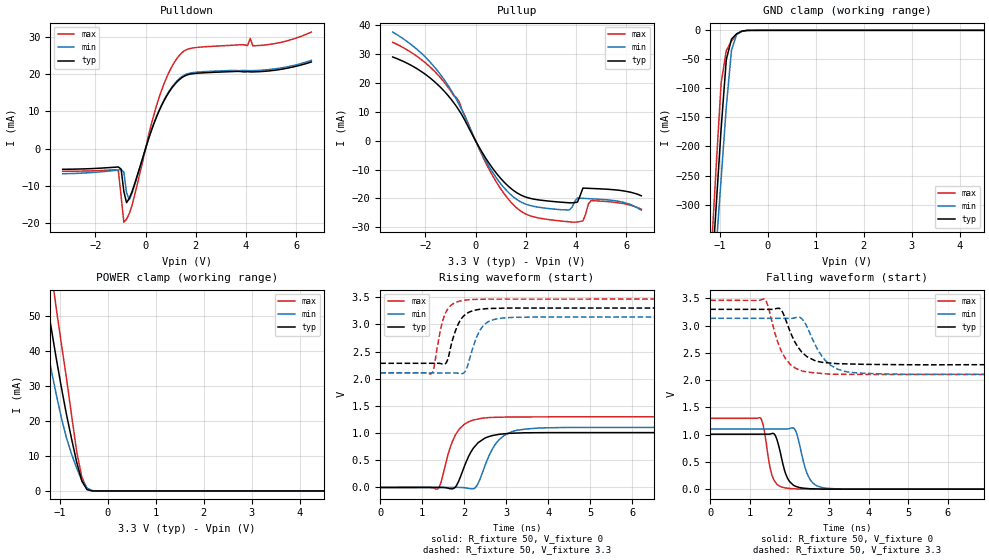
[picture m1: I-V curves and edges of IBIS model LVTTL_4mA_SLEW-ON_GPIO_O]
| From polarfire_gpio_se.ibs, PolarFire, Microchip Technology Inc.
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|   Model LVTTL_4mA_SLEW-ON_GPIO_O
[Model]   LVTTL_4mA_SLEW-ON_GPIO_O
Model_type   Output
Polarity   Non-Inverting
Enable   Active-High
Vmeas =   1.65
Cref =   5p
Rref =   1M
|   typ   min   max
C_comp_pullup   2.605e-12   2.605e-12   2.76e-12
C_comp_pulldown  2.605e-12   2.605e-12   2.76e-12
[Temperature Range]  25C   100C   -40C
[Voltage Range]  3.3   3.135   3.465
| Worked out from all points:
|   slope of the pulldown table from 0 to 0.495 V, typ, clamps not added: 52.5 ohm
|   slope of the pullup table from 0 to 0.495 V, typ, clamps not added: 68.4 ohm
|   GND clamp passes 1 mA (typ) near -0.51 V on its own axis
|   POWER clamp passes 1 mA (typ) near -0.46 V on its own axis
|   rising waveform, R_fixture 50, V_fixture 0: 20-80 % time 399ps typ, 429ps min, 348ps max; typ from 0 V to 1.01 V
|   rising waveform, R_fixture 50, V_fixture 3.3: 20-80 % time 275ps typ, 299ps min, 229ps max; typ from 2.28 V to 3.3 V
|   falling waveform, R_fixture 50, V_fixture 0: 20-80 % time 226ps typ, 254ps min, 186ps max; typ from 1.01 V to 0 V
|   falling waveform, R_fixture 50, V_fixture 3.3: 20-80 % time 444ps typ, 505ps min, 403ps max; typ from 3.3 V to 2.28 V
[GND Clamp]
| Voltage   I(typ)   I(min)   I(max)
-3.3V     -3.213A    -2.957A    -3.542A
-1.191V   -450mA     -505.3mA   -401.1mA
-1.083V   -310.2mA   -380.8mA   -242.7mA
-974.5mV  -170.4mA   -256.4mA   -91.54mA
-866.2mV  -50.48mA   -132.2mA   -34.88mA
-758mV    -15.08mA   -34.24mA   -18.56mA
-649.7mV  -5.883mA   -6.714mA   -7.365mA
-541.4mV  -1.389mA   -1.466mA   -1.709mA
-433.1mV  -123uA     -170uA     -145.5uA
-108.3mV  -6.015nA   -17.98nA   -17.62nA
6.6V      0A         0A         0A
[POWER Clamp]
| Voltage   I(typ)   I(min)   I(max)
-3.3V     320.3mA    266.4mA    379mA
-1.624V   89.11mA    69.3mA     113.8mA
-1.408V   67.23mA    51.37mA    87.82mA
-1.299V   57.08mA    43.14mA    75.67mA
-1.191V   47.51mA    35.38mA    63.94mA
-1.083V   38.51mA    28.09mA    52.96mA
-866.2mV  22.14mA    15.36mA    32.61mA
-649.7mV  8.213mA    6.528mA    11.28mA
-541.4mV  2.791mA    3.019mA    3.88mA
-433.1mV  359.8uA    815.7uA    615.5uA
-216.6mV  159.8nA    4.578uA    2.748uA
6.6V      0A         0A         0A
[Pullup]
| Voltage   I(typ)   I(min)   I(max)
-3.3V     29.06mA    37.69mA    34.14mA
-1.841V   22mA       27.59mA    25.83mA
-758mV    11.88mA    14.29mA    14.95mA
618.8mV   -8.81mA    -10.12mA   -11.17mA
1.238V    -15.2mA    -17.29mA   -19.51mA
1.856V    -19.03mA   -21.44mA   -24.7mA
3.733V    -21.5mA    -23.97mA   -28.1mA
3.95V     -21.43mA   -20.97mA   -28.22mA
4.058V    -21.25mA   -19.85mA   -28.14mA
4.275V    -16.4mA    -19.95mA   -27.77mA
4.599V    -16.52mA   -20.11mA   -20.73mA
6.6V      -19.07mA   -24.04mA   -23.71mA
[Pulldown]
| Voltage   I(typ)   I(min)   I(max)
-3.3V     -5.571mA   -6.764mA   -6.091mA
-1.083V   -4.968mA   -5.761mA   -6.034mA
-974.5mV  -5.532mA   -5.644mA   -12.81mA
-866.2mV  -11.51mA   -6.329mA   -19.8mA
-758mV    -14.57mA   -11.89mA   -19mA
-649.7mV  -13.39mA   -13.75mA   -17.48mA
515.6mV   9.754mA    9.89mA     13.24mA
928.1mV   15.09mA    15.32mA    20.43mA
1.444V    19.03mA    19.29mA    25.73mA
4.166V    20.59mA    20.9mA     29.56mA
4.924V    20.85mA    21.23mA    27.96mA
6.6V      23.25mA    23.69mA    31.28mA
[Ramp]
dV/dt_r   0.605268/0.399125n  0.662241/0.428734n  0.779561/0.348269n
dV/dt_f   0.609728/0.443928n  0.616346/0.504767n  0.815859/0.403227n
R_load = 50
[Rising Waveform]
R_fixture = 50
V_fixture = 0
V_fixture_min = 0
V_fixture_max = 0
| Time   V(typ)   V(min)   V(max)
0s        84.25nV    61.34nV    248.1nV
1.363ns   830uV      715.2uV    -27.65mV
1.447ns   942.9uV    759.2uV    100.9mV
1.653ns   -21.41mV   867.3uV    707.2mV
1.785ns   4.621mV    936.6uV    961.7mV
2.241ns   745.2mV    -15.83mV   1.244V
2.431ns   876.6mV    270.7mV    1.275V
2.759ns   967.5mV    814.4mV    1.29V
3.255ns   1.001V     1.053V     1.296V
10ns      1.009V     1.104V     1.299V
[Rising Waveform]
R_fixture = 50
V_fixture = 3.3
V_fixture_min = 3.135
V_fixture_max = 3.465
| Time   V(typ)   V(min)   V(max)
0s        2.284V     2.108V     2.105V
1.222ns   2.284V     2.107V     2.098V
1.279ns   2.284V     2.107V     2.209V
1.443ns   2.278V     2.107V     2.929V
1.543ns   2.274V     2.107V     3.191V
1.834ns   2.969V     2.103V     3.413V
2.015ns   3.175V     2.129V     3.446V
2.369ns   3.277V     2.885V     3.461V
2.769ns   3.295V     3.1V       3.464V
10ns      3.3V       3.135V     3.465V
[Falling Waveform]
R_fixture = 50
V_fixture = 0
V_fixture_min = 0
V_fixture_max = 0
| Time   V(typ)   V(min)   V(max)
0s        1.009V     1.104V     1.299V
1.267ns   1.009V     1.104V     1.305V
1.352ns   1.009V     1.104V     1.113V
1.569ns   1.022V     1.104V     232.2mV
1.686ns   901.7mV    1.104V     90.54mV
1.894ns   303.1mV    1.104V     22.71mV
2.141ns   57.55mV    1.091V     6.532mV
2.475ns   10.44mV    237.1mV    1.336mV
2.812ns   1.974mV    32.15mV    588.3uV
10ns      663.1nV    1.835uV    209.8nV
[Falling Waveform]
R_fixture = 50
V_fixture = 3.3
V_fixture_min = 3.135
V_fixture_max = 3.465
| Time   V(typ)   V(min)   V(max)
0s        3.3V       3.135V     3.465V
1.375ns   3.299V     3.134V     3.486V
1.448ns   3.299V     3.134V     3.38V
1.632ns   3.309V     3.134V     2.865V
1.799ns   3.282V     3.134V     2.525V
2.017ns   2.892V     3.134V     2.292V
2.314ns   2.513V     3.125V     2.168V
2.898ns   2.322V     2.367V     2.118V
3.453ns   2.299V     2.151V     2.107V
10ns      2.284V     2.108V     2.105V
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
